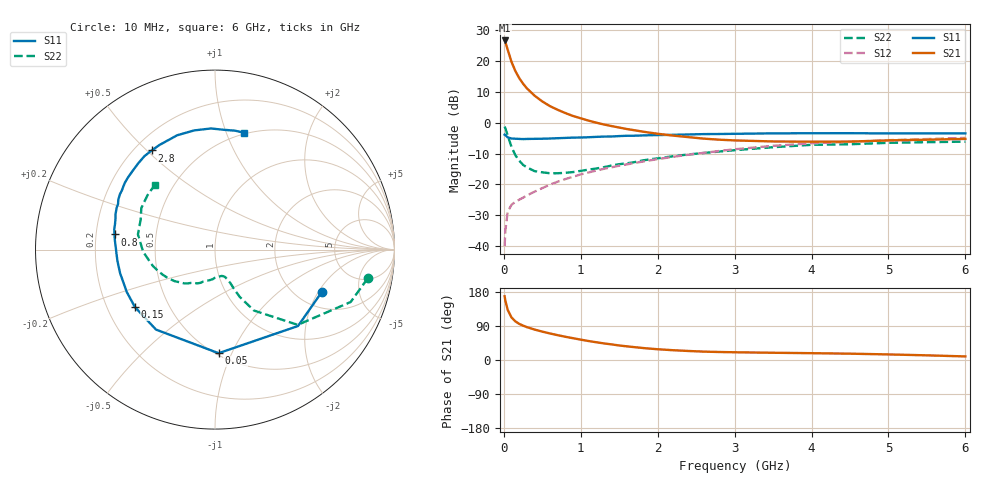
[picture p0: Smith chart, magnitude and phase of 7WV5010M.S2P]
! Infineon Technologies  Discrete & RF Semiconductors
! BFS17W
! Si NPN RF Bipolar Junction Transistor in SOT323
! VCE = 0.5 V  IC = 10 mA
! Common Emitter S-Parameters:  August  1999
# GHz  S  MA  R  50
!  f  S11  S21  S12  S22
! GHz  MAG  ANG  MAG  ANG  MAG  ANG  MAG  ANG
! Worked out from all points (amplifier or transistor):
!   36 points, 10 MHz to 6 GHz, reference 50 ohm
!   highest |S21| = 26.6 dB at 10 MHz (marker M1)
!   |S21| within 3 dB of that: start of sweep to 50.06 MHz
!   unconditionally stable (mu >= 1): 170.6 MHz to end of sweep
!   at 250 MHz: K = 1.31, MAG = 15.1 dB, |S12| = -24.3 dB
!   at 1.4 GHz: K = 1.87, MAG = 1.3 dB, |S12| = -14.5 dB
!   at 6 GHz: K = 1.16, MAG = -2.6 dB, |S12| = -4.9 dB
!   S11 on the Smith chart (normalised r, x): 10 MHz: 2.67, -2.15; 50 MHz: 0.52, -0.89; 150 MHz: 0.32, -0.29; 800 MHz: 0.28, +0.07; 2.8 GHz: 0.27, +0.52; 6 GHz: 0.49, +1.16
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0.01  0.6398 -21.8  21.43 168.2  0.01 78.0  0.8662 -10.6
0.02  0.6287 -42.6  20.25 156.5  0.0179 71.8  0.8105 -21.1
0.05  0.5775 -88.0  15.18 132.4  0.0363 51.9  0.623 -42.3
0.1  0.5538 -126.4  9.628 112.2  0.0468 41.0  0.4029 -57.4
0.15  0.5492 -144.3  6.842 101.9  0.0523 39.1  0.2972 -62.4
0.2  0.5454 -154.3  5.264 95.4  0.0566 40.7  0.2423 -64.2
0.25  0.5421 -161.0  4.279 90.7  0.061 42.8  0.2073 -65.3
0.3  0.5448 -165.9  3.588 86.7  0.0663 45.0  0.1886 -66.4
0.4  0.547 -173.0  2.732 80.3  0.0763 48.9  0.164 -69.6
0.5  0.5496 -177.8  2.207 74.9  0.0872 51.7  0.1571 -71.6
0.6  0.5537 178.2  1.85 70.0  0.0992 53.7  0.1515 -75.5
0.8  0.5662 171.4  1.429 61.3  0.122 55.8  0.1542 -86.1
0.9  0.5729 168.5  1.282 57.5  0.1331 56.5  0.1585 -91.3
1.1  0.5807 162.7  1.079 50.1  0.1561 56.7  0.1735 -100.4
1.3  0.5953 157.1  0.934 43.8  0.1788 56.4  0.1901 -110.3
1.6  0.6128 149.9  0.788 36.0  0.2112 55.5  0.2194 -122.2
2.2  0.6354 135.9  0.617 25.8  0.2796 52.6  0.2857 -142.0
2.8  0.6551 122.5  0.53 21.1  0.3475 47.4  0.3405 -160.1
3.5  0.671 108.3  0.496 19.1  0.4224 39.7  0.4002 -178.1
4.5  0.6753 91.9  0.494 16.7  0.4879 28.1  0.4468 157.9
5.5  0.672 80.4  0.53 12.3  0.5426 18.8  0.483 141.0
6  0.6709 75.9  0.546 9.4  0.5675 14.3  0.4927 132.9
